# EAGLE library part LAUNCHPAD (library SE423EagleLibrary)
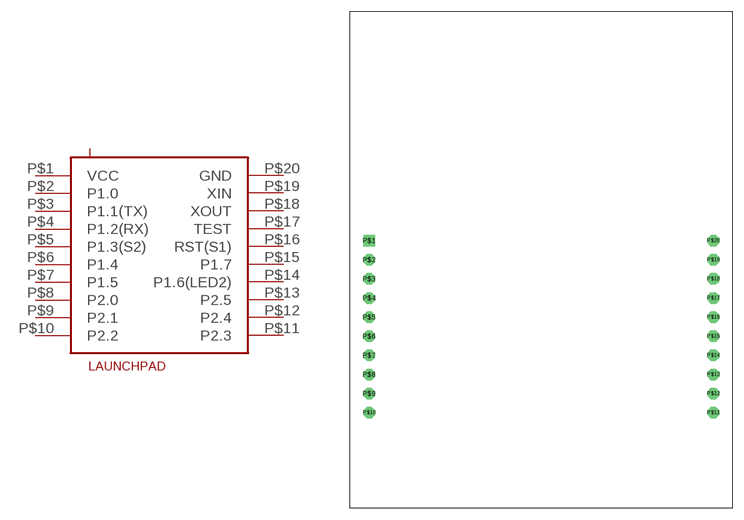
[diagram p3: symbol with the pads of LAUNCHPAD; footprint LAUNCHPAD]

Designator prefix L

## LAUNCHPAD  [LAUNCHPAD]
P$1  VCC
P$2  P1.0
P$3  P1.1(TX)
P$4  P1.2(RX)
P$5  P1.3(S2)
P$6  P1.4
P$7  P1.5
P$8  P2.0
P$9  P2.1
P$10  P2.2
P$11  P2.3
P$12  P2.4
P$13  P2.5
P$14  P1.6(LED2)
P$15  P1.7
P$16  RST(S1)
P$17  TEST
P$18  XOUT
P$19  XIN
P$20  GND

## Footprint LAUNCHPAD (pad centres in mm)
drill 1.016 square: P$1 0,0
drill 1.016 octagon: P$2 0,-2.54; P$3 0,-5.08; P$4 0,-7.62; P$5 0,-10.16; P$6 0,-12.7; P$7 0,-15.24; P$8 0,-17.78; P$9 0,-20.32; P$10 0,-22.86; P$11 45.72,-22.86; P$12 45.72,-20.32; P$13 45.72,-17.78; P$14 45.72,-15.24; P$15 45.72,-12.7; P$16 45.72,-10.16; P$17 45.72,-7.62; P$18 45.72,-5.08; P$19 45.72,-2.54; P$20 45.72,0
